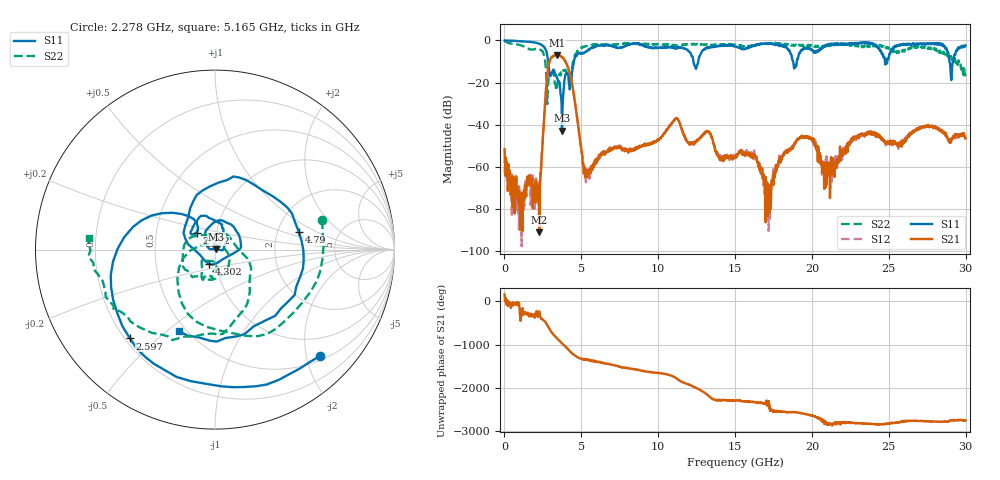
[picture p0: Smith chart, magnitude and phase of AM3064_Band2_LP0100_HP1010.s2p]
# Hz S DB R 50.0
!freq dBS11 angS11 dBS21 angS21 dBS12 angS12 dBS22 angS22
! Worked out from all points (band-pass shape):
!   1600 points, 10 MHz to 29.98 GHz, reference 50 ohm
!   highest |S21| = -6.86 dB at 3.403 GHz (marker M1); lowest = -91.0 dB at 2.278 GHz (marker M2)
!   |S21| within 3 dB of the highest: 2.935 GHz to 3.952 GHz (1.017 GHz wide, 29.5 % of centre)
!   lowest |S11| = -42.8 dB at 3.74 GHz (marker M3), VSWR 1.01, Z = 50.7 + j0.147 ohm
!   |S11| at or under -10 dB: 2.84 GHz to 4.506 GHz (1.666 GHz wide, 45.4 % of centre); 12.29 GHz to 12.6 GHz (308.9 MHz wide, 2.48 % of centre); 28.94 GHz to 29.2 GHz (258.1 MHz wide, 0.888 % of centre)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
!   |S22| runs from -30.2 to -0.2 dB; largest |S21 - S12| = 0.016
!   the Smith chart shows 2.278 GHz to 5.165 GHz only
!   S11 on the Smith chart (normalised r, x): 2.278 GHz: 0.58, -2.27; 2.597 GHz: 0.22, -0.41; 2.972 GHz: 0.80, +0.16; 4.302 GHz: 0.92, -0.15; 4.79 GHz: 2.63, +0.67; 5.165 GHz: 0.45, -0.55
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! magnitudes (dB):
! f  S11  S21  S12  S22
! 10 MHz  0.0  -51.6  -59.7  -0.2
! 1.078 GHz  -0.4  -79.1  -88.6  -2.4
! 2.278 GHz  -1.6  -91.0  -67.9  -4.2
! 2.597 GHz  -3.3  -34.3  -34.4  -7.7
! 2.972 GHz  -17.1  -9.2  -9.1  -16.6
! 3.403 GHz  -17.4  -6.9  -7.1  -23.3
! 3.74 GHz  -42.8  -8.0  -7.8  -14.9
! 4.302 GHz  -21.2  -17.1  -17.1  -19.3
! 4.79 GHz  -6.4  -40.3  -40.0  -4.7
! 5.015 GHz  -6.4  -51.9  -52.8  -3.7
! 5.165 GHz  -6.1  -63.1  -59.6  -3.0
! 10 GHz  -3.5  -46.9  -47.0  -1.8
! 11.2 GHz  -3.7  -37.0  -37.0  -2.3
! 15 GHz  -2.6  -55.5  -55.5  -2.0
! 16.28 GHz  -2.3  -54.4  -56.3  -2.4
! 17.2 GHz  -1.6  -68.4  -76.6  -1.6
! 17.99 GHz  -2.7  -55.1  -54.9  -1.5
! 19.99 GHz  -4.3  -46.6  -47.1  -2.2
! 20.82 GHz  -2.8  -57.8  -56.7  -2.4
! 22.84 GHz  -1.4  -46.0  -47.4  -2.2
! 25 GHz  -8.2  -47.8  -48.9  -3.4
! 29.98 GHz  -2.3  -46.5  -46.3  -15.8
